// TwinCAT 3 PLC project homing
// ProgramVersion: 3.1.4020.4
// libraries:
//   Tc2_MC2, * (Beckhoff Automation GmbH)
//   Tc2_Standard, * (Beckhoff Automation GmbH)
//   Tc2_System, * (Beckhoff Automation GmbH)
//   Tc3_Module, * (Beckhoff Automation GmbH)
// project tree:
//   / GlobalTextList.TcGTLO, PlcTask.TcTTO, Visualization Manager.TcVMO
//   POUs/ MAIN.TcPOU
//   VISUs/ hmi.TcVIS
// real-time tasks:
//   TASK PlcTask: cycle T#10ms, priority 20, ADS port 350
// motion (NC):
//   TASK NC-Task 1 SAF: cycle T#2ms, priority 4, ADS port 501
//   TASK NC-Task 1 SVB: cycle T#10ms, priority 8, ADS port 511
//   AXIS Axis 1 (id 1)
//     Dynamic: Acceleration=660.96, Deceleration=660.96, Jerk=1908.05, DelayTime=0.008
//     Velo: RefSync=5, SlowManual=50, FastManual=200, Maximum=432
//     OtherSettings: AllowMotionCmdToSlave=true
//     encoder EncType=4
//       EncPara: ScaleFactorNumerator=360, ScaleFactorDenominator=3200, MaxCount=#x0000ffff
//         Inc: RefMode=1, RefSoftSyncMask=#x0000ffff
//     drive DrvType=5
//       Analog: VeloReferenz=360
//       TimeComp: TaskDelayCycles=1
//     controller CtrType=3
//       CtrPara: PriorControlFactor=1
//         PID: PosKp=2.5, VeloKp=1, VeloTn=0.07
//         Observer: BandWidth=20
// I/O:
//   DEVICE Device 1 (EtherCAT), AmsNetId 5.12.242.16.2.1
//     Term 1 (EK1200) [EK1200-5000 EtherCAT Power supply (2A E-Bus)]
//       Term 2 (EL1004) [EL1004 4Ch. Dig. Input 24V, 3ms]
//       Term 3 (EL2032) [EL2032 2Ch. Dig. Output 24V, 2A Diag]
//       Term 4 (EL2521) [EL2521 1Ch. Pulse Train Output]
//       Term 5 (EL9011) [EL9011 End Terminal]
// variable links:
//   NC-Task 1 SAF/Axes/Axis 1 <-> Device 1 (EtherCAT)/Term 1 (EK1200)/Term 4 (EL2521)
//     Drive/Inputs/In/nState1 @bit 6 <-> PTO Status/Status/Error
//     Drive/Inputs/In/nState1 @bit 1 <-> PTO Status/Status/Ramp active
//     Drive/Inputs/In/nState1 <-> PTO Status/Status/Sel. Ack/End counter
//     Drive/Inputs/In/nState1 @bit 4 <-> PTO Status/Status/Status of input target
//     Drive/Inputs/In/nState1 @bit 5 <-> PTO Status/Status/Status of input zero
//     Drive/Inputs/In/nState4 @bit 1 <-> WcState/InputToggle
//     Drive/Inputs/In/nState4 <-> WcState/WcState
//     Drive/Outputs/Out/nCtrl1 @bit 1 <-> PTO Control/Control/Disable ramp
//     Drive/Outputs/Out/nCtrl1 <-> PTO Control/Control/Frequency select
//     Drive/Outputs/Out/nCtrl1 @bit 2 <-> PTO Control/Control/Go counter
//     Drive/Outputs/Out/nDataOut1[0] <-> PTO Control/Frequency value
//     Enc/Inputs/In/nDataIn1[0] <-> ENC Status compact/Counter value
//     Enc/Inputs/In/nState1 @bit 4 <-> ENC Status compact/Status/Counter overflow
//     Enc/Inputs/In/nState1 @bit 3 <-> ENC Status compact/Status/Counter underflow
//     Enc/Inputs/In/nState1 @bit 2 <-> ENC Status compact/Status/Set counter done
//     Enc/Inputs/In/nState4 @bit 1 <-> WcState/InputToggle
//     Enc/Inputs/In/nState4 <-> WcState/WcState
//     Enc/Outputs/Out/nCtrl1 @bit 2 <-> ENC Control compact/Control/Set counter
//     Enc/Outputs/Out/nDataOut1[0] <-> ENC Control compact/Set counter value
//   homing/homing Instance <-> Device 1 (EtherCAT)/Term 1 (EK1200)/Term 2 (EL1004)
//     PlcTask Inputs/MAIN.sensor <-> Channel 1/Input
//   homing/homing Instance <-> NC-Task 1 SAF/Axes/Axis 1
//     PlcTask Inputs/MAIN.el2521_axis.NcToPlc <-> Outputs/ToPlc
//     PlcTask Outputs/MAIN.el2521_axis.PlcToNc <-> Inputs/FromPlc

CONFIGURATION homing
    RESOURCE PLC ON TwinCAT3
        TASK PlcTask(INTERVAL := T#10ms, PRIORITY := 20);
        PROGRAM MAIN WITH PlcTask : MAIN;
    END_RESOURCE
END_CONFIGURATION

// ---- POUs/MAIN.TcPOU
PROGRAM MAIN
VAR
	el2521_axis:	axis_ref;
	el2521_power:	mc_power;
	el2521_home:	mc_home;
	home_do: BOOL;			(*用HMI中的开关代替*)
	sensor AT %I*: BOOL;	(*EL1004的1通道*)
END_VAR

//使能
el2521_power(Axis:=el2521_axis , Enable:= TRUE, Enable_Positive:=TRUE , Enable_Negative:=TRUE ,  );
//找原点
el2521_home(Axis:=el2521_axis , Execute:= home_do, Position:=0 ,bCalibrationCam:=sensor ,  );

END_PROGRAM

// ---- GlobalTextList.TcGTLO
TEXTLIST GlobalTextList
  0 = 'axis_pos:%.2f'
END_TEXTLIST

// ---- VISUs/hmi.TcVIS
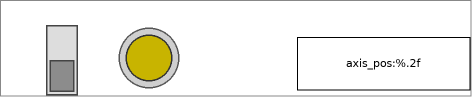
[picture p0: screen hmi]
VISUALIZATION hmi  // 472x97
    DipSwitch (27,25 70x70), variable: MAIN.home_do, behaviour: TOGGLE, style: Switch-DipSwitch-Gray
    Lamp1 (114,23 70x70), variable: MAIN.sensor, style: Lamp-Lamp1-Yellow
    Rectangle (297,37 173x53), "axis_pos:%.2f", text variable: MAIN.el2521_axis.NcToPlc.ActPos
END_VISUALIZATION
